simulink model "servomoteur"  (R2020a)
settings: Solver=VariableStepAuto  StartTime=0.0  StopTime=0.04  RelTol=1e-3
model workspace (MAT data in the model file):
  rp_cyclique_esp = 20

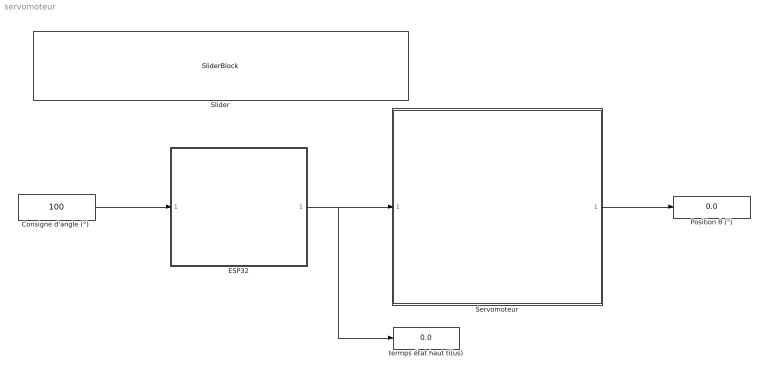
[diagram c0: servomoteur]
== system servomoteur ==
  "Consigne d'angle (°) " : Constant  Value=100
  ESP32 : Subsystem
  Position θ (°) : Display
  Servomoteur : Subsystem
  Slider : SliderBlock  ScaleMin=1  ScaleMax=180  TickInterval=10
  termps état haut ti(us) : Display
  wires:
  "Consigne d'angle (°) "/1 -> ESP32/1(In1)
  ESP32/1(Out1) -> Servomoteur/1(In1), termps état haut ti(us)/1
  Servomoteur/1(Out1) -> Position θ (°)/1

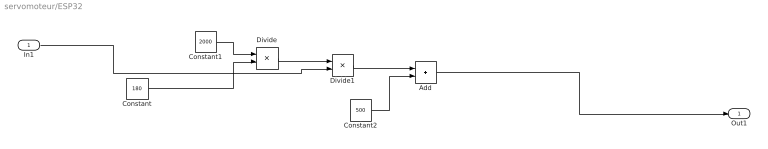
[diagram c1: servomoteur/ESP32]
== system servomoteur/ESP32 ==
  In1 : Inport
  Add : Sum
  Constant : Constant  Value=180
  Constant1 : Constant  Value=2000
  Constant2 : Constant  Value=500
  Divide : Product  Inputs=*/
  Divide1 : Product  Inputs=**
  Out1 : Outport  VectorParamsAs1DForOutWhenUnconnected=off
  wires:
  Constant/1 -> Divide/2
  Constant1/1 -> Divide/1
  Divide/1 -> Divide1/1
  Divide1/1 -> Add/1
  Constant2/1 -> Add/2
  In1/1 -> Divide1/2
  Add/1 -> Out1/1

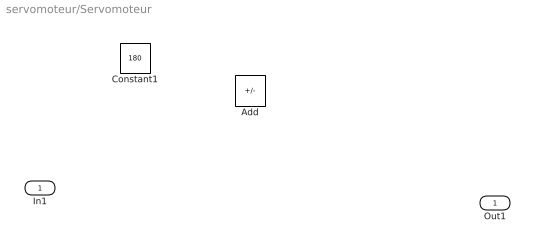
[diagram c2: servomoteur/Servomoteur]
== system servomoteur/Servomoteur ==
  In1 : Inport
  Add : Sum  Inputs=+-
  Constant1 : Constant  Value=180
  Out1 : Outport  VectorParamsAs1DForOutWhenUnconnected=off
